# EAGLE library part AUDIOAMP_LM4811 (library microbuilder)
LM4811 - Dual 105mW Headphone Amplifier with Digital Volume Control Digikey: MSOP-10 - LM4811MMCT-ND
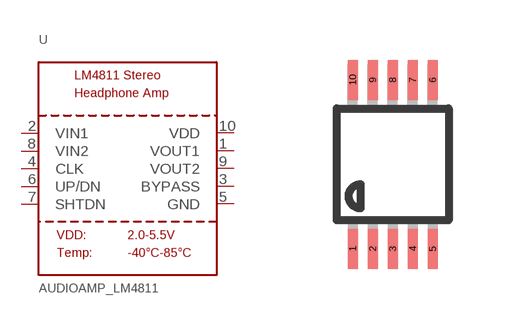
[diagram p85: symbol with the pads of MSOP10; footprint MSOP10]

Designator prefix U

## AUDIOAMP_LM4811  [MSOP10]
1  VOUT1
2  VIN1
3  BYPASS
4  CLK
5  GND
6  UP/DN
7  SHTDN
8  VIN2
9  VOUT2
10  VDD

## Footprint MSOP10 (pad centres in mm)
10-Lead Mini Small Outline Package [MSOP]
smd 0.25 x 1: 1 -1,-2.113; 2 -0.5,-2.113; 3 0,-2.113; 4 0.5,-2.113; 5 1,-2.113; 6 1,2.113; 7 0.5,2.113; 8 0,2.113; 9 -0.5,2.113; 10 -1,2.113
